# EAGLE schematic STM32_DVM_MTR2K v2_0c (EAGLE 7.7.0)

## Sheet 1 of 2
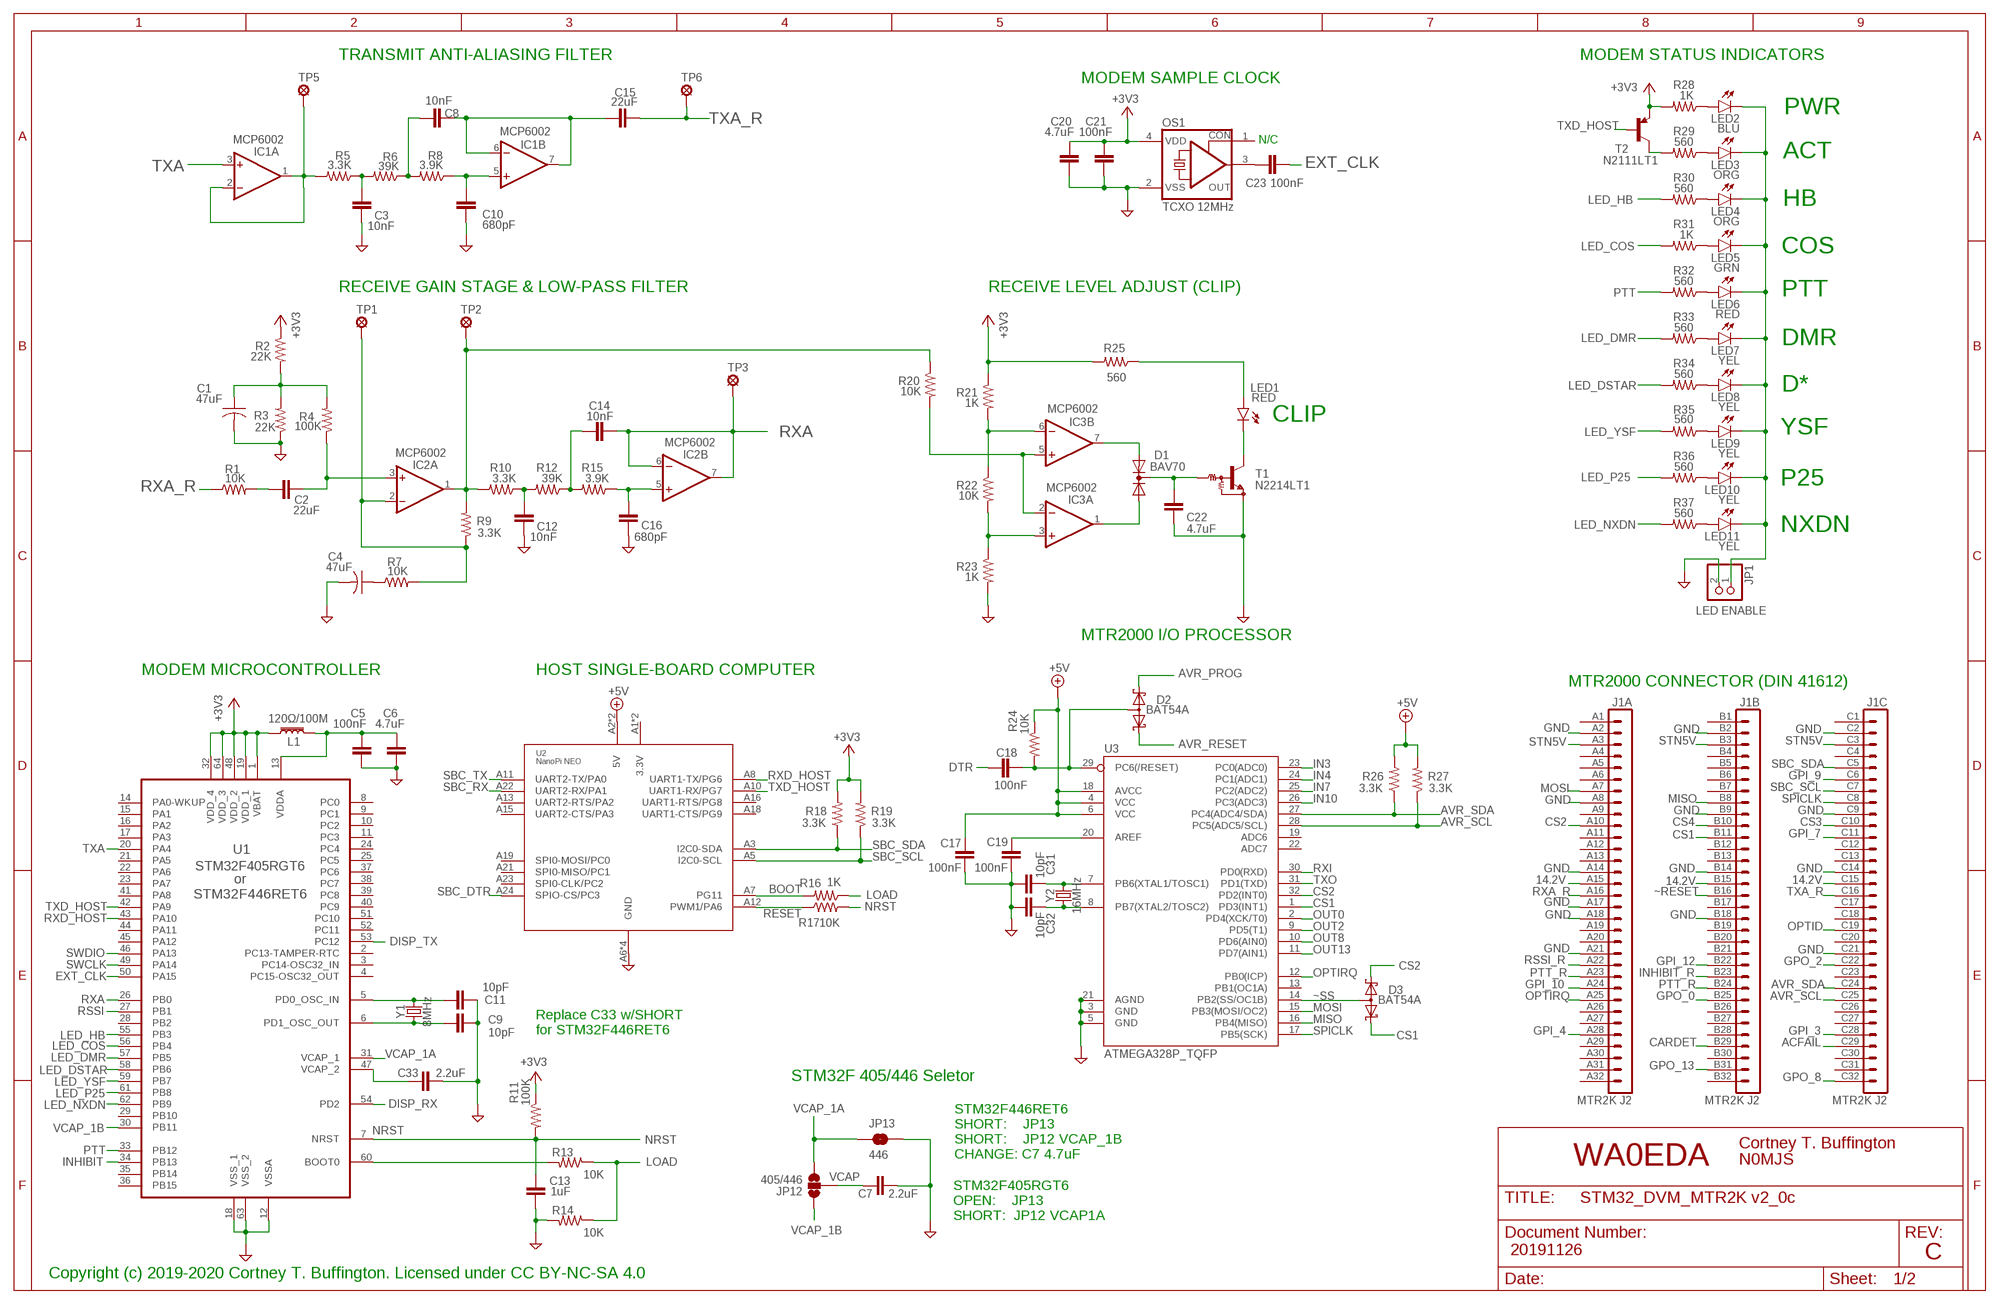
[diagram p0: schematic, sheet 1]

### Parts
C1  47uF  C-USC1210  [C1210]
C2  22uF  C-EUC1210  [C1210]
C3  10nF  C-EUC0805  [C0805]
C4  47uF  C-USC1210  [C1210]
C5  100nF  C-EUC0805  [C0805]
C6  4.7uF  C-EUC0805  [C0805]
C7  2.2uF  C-EUC0805  [C0805]
C8  10nF  C-EUC0805  [C0805]
C9  10pF  C-EUC0805  [C0805]
C10  680pF  C-EUC0805  [C0805]
C11  10pF  C-EUC0805  [C0805]
C12  10nF  C-EUC0805  [C0805]
C13  1uF  C-EUC0805  [C0805]
C14  10nF  C-EUC0805  [C0805]
C15  22uF  C-EUC1210  [C1210]
C16  680pF  C-EUC0805  [C0805]
C17  100nF  C-EUC0805  [C0805]
C18  100nF  C-EUC0805  [C0805]
C19  100nF  C-EUC0805  [C0805]
C20  4.7uF  C-EUC0805  [C0805]
C21  100nF  C-EUC0805  [C0805]
C22  4.7uF  C-EUC0805  [C0805]
C23  100nF  C-EUC0805  [C0805]
C31  10pF  C-EUC0805  [C0805]
C32  10pF  C-EUC0805  [C0805]
C33  2.2uF  C-EUC0805  [C0805]
D1  BAV70  DIODE_AC-CA_  [SOT23C]
D2  BAT54A  [SOT23]
D3  BAT54A  [SOT23]
IC1  MCP6002  TL082D  [SO08]
IC2  MCP6002  TL082D  [SO08]
IC3  MCP6002  TL082D  [SO08]
J1  MTR2K J2  VG96-3  [VG96]
JP1  LED ENABLE  PINHD-1X2  [1X02]
JP12  405/446  JUMPER-SMT_3_NO_NO-SILK  [SMT-JUMPER_3_NO_NO-SILK]
JP13  446  JUMPER-SMT_2_NO_NO-SILK  [SMT-JUMPER_2_NO_NO-SILK]
L1  120Ω/100M  FERRITE_BEAD-0603  [0603]
LED1  RED  LED0603  [LED-0603]
LED2  BLU  LED0603  [LED-0603]
LED3  ORG  LED0603  [LED-0603]
LED4  ORG  LED0603  [LED-0603]
LED5  GRN  LED0603  [LED-0603]
LED6  RED  LED0603  [LED-0603]
LED7  YEL  LED0603  [LED-0603]
LED8  YEL  LED0603  [LED-0603]
LED9  YEL  LED0603  [LED-0603]
LED10  YEL  LED0603  [LED-0603]
LED11  YEL  LED0603  [LED-0603]
OS1  TCXO 12MHz  OSC-OE-CFPS-9  [5.2X3.4-4-PAD]
R1  10K  R-US_R0805  [R0805]
R2  22K  R-US_R0805  [R0805]
R3  22K  R-US_R0805  [R0805]
R4  100K  R-US_R0805  [R0805]
R5  3.3K  R-US_R0805  [R0805]
R6  39K  R-US_R0805  [R0805]
R7  10K  R-US_R0805  [R0805]
R8  3.9K  R-US_R0805  [R0805]
R9  3.3K  R-US_R0805  [R0805]
R10  3.3K  R-US_R0805  [R0805]
R11  100K  R-US_R0805  [R0805]
R12  39K  R-US_R0805  [R0805]
R13  10K  R-US_R0805  [R0805]
R14  10K  R-US_R0805  [R0805]
R15  3.9K  R-US_R0805  [R0805]
R16  1K  R-US_R0805  [R0805]
R17  10K  R-US_R0805  [R0805]
R18  3.3K  R-US_R0805  [R0805]
R19  3.3K  R-US_R0805  [R0805]
R20  10K  R-US_R0805  [R0805]
R21  1K  R-US_R0805  [R0805]
R22  10K  R-US_R0805  [R0805]
R23  1K  R-US_R0805  [R0805]
R24  10K  R-US_R0805  [R0805]
R25  560  R-US_R0805  [R0805]
R26  3.3K  R-US_R0805  [R0805]
R27  3.3K  R-US_R0805  [R0805]
R28  1K  R-US_R0805  [R0805]
R29  560  R-US_R0805  [R0805]
R30  560  R-US_R0805  [R0805]
R31  1K  R-US_R0805  [R0805]
R32  560  R-US_R0805  [R0805]
R33  560  R-US_R0805  [R0805]
R34  560  R-US_R0805  [R0805]
R35  560  R-US_R0805  [R0805]
R36  560  R-US_R0805  [R0805]
R37  560  R-US_R0805  [R0805]
T1  N2214LT1  MUN2211T1-NPN_DRIVER-SC59-BEC  [SC59-BEC]
T2  N2111LT1  MMUN2111LT1-PNP-SC59-BEC  [SC59-BEC]
TP1  MCS10B  [MCS10B]
TP2  MCS10B  [MCS10B]
TP3  MCS10B  [MCS10B]
TP5  MCS10B  [MCS10B]
TP6  MCS10B  [MCS10B]
U1  STM32F405RGT6  [QFP50P1200X1200X160-64N]
U2  NanoPi NEO  NANOPI-NEO_MINIMALMINIMAL  [NANOPI-NEO]
U3  ATMEGA328P_TQFP  [TQFP32-08]
Y1  8MHz  CRYSTALSMD-3.2X2.5  [CRYSTAL-SMD-3.2X2.5MM]
Y2  16MHz  CRYSTALSMD-3.2X2.5  [CRYSTAL-SMD-3.2X2.5MM]

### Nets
14.2V: J1.A15 J1.B15 J1.C15 ; also sheet 2
+3V3: C20.2 C21.2 L1.1 OS1.4(VDD) R2.1 R11.1 R18.2 R19.2 R21.1 R25.2 R28.2 T2.E U1.1(VBAT) U1.19(VDD_1) U1.32(VDD_4) U1.48(VDD_2) U1.64(VDD_3) ; also sheet 2
+5V: C17.2 R24.1 R26.2 R27.2 U2.A2(5V) U2.A4(5V) U3.4(VCC) U3.6(VCC) U3.18(AVCC) ; also sheet 2
ACFAIL: J1.C29
AREF: C19.2 U3.20(AREF)
AVR_PROG: D2.1(K1) ; also sheet 2
AVR_RESET: D2.2(K2) ; also sheet 2
AVR_SCL: J1.C25 R27.1 U3.28(PC5(ADC5/SCL))
AVR_SDA: J1.C24 R26.1 U3.27(PC4(ADC4/SDA))
BOOT: R16.2 U2.A7(PG11) ; also sheet 2
BOOT0: R13.2 U1.60(BOOT0)
CARDET: J1.B29
CS1: D3.2(K2) J1.B11 U3.1(PD3(INT1))
CS2: D3.1(K1) J1.A10 U3.32(PD2(INT0))
CS3: J1.C10
CS4: J1.B10
DISP_RX: U1.54(PD2) ; also sheet 2
DISP_TX: U1.53(PC12) ; also sheet 2
DTR: C18.2 ; also sheet 2
EXT_CLK: C23.2 U1.50(PA15)
GND: C1.2 C3.2 C4.2 C5.1 C6.1 C7.1 C9.2 C10.2 C11.2 C12.2 C13.2 C16.2 C17.1 C19.1 C20.1 C21.1 C22.2 C31.2 C32.2 C33.1 J1.A2 J1.A8 J1.A14 J1.A17 J1.A18 J1.A21 J1.B2 J1.B9 J1.B14 J1.B18 J1.C2 J1.C9 J1.C14 J1.C21 JP1.2 JP13.2 OS1.2(VSS) R3.1 R14.2 R23.2 T1.E U1.12(VSSA) U1.18(VSS_1) U1.63(VSS_2) U2.A6(GND) U2.A9(GND) U2.A14(GND) U2.A20(GND) U3.3(GND) U3.5(GND) U3.21(AGND) ; also sheet 2
GPI_3: J1.C28 ; also sheet 2
GPI_4: J1.A28 ; also sheet 2
GPI_7: J1.C11 ; also sheet 2
GPI_9: J1.C6
GPI_10: J1.A24 ; also sheet 2
GPI_12: J1.B22
GPO_0: J1.B25 ; also sheet 2
GPO_2: J1.C22 ; also sheet 2
GPO_8: J1.C32 ; also sheet 2
GPO_13: J1.B31 ; also sheet 2
IN3: U3.23(PC0(ADC0)) ; also sheet 2
IN4: U3.24(PC1(ADC1)) ; also sheet 2
IN7: U3.25(PC2(ADC2)) ; also sheet 2
IN10: U3.26(PC3(ADC3)) ; also sheet 2
INHIBIT: U1.34(PB13) ; also sheet 2
INHIBIT_R: J1.B23 ; also sheet 2
LED_COS: R31.2 U1.56(PB4)
LED_DMR: R33.2 U1.57(PB5)
LED_DSTAR: R34.2 U1.58(PB6)
LED_HB: R30.2 U1.55(PB3)
LED_NXDN: R37.2 U1.62(PB9)
LED_P25: R36.2 U1.61(PB8)
LED_YSF: R35.2 U1.59(PB7)
LOAD: R13.1 R14.1 R16.1 ; also sheet 2
MISO: J1.B8 U3.16(PB4(MISO)) ; also sheet 2
MOSI: J1.A7 U3.15(PB3(MOSI/OC2)) ; also sheet 2
N$1: C23.1 OS1.3(OUT)
N$2: C2.2 R1.2
N$5: C4.1 R7.1
N$10: C8.2 C15.2 IC1.6(B:-IN) IC1.7(B:OUT)
N$11: C11.1 U1.5(PD0_OSC_IN) Y1.3
N$12: C9.1 U1.6(PD1_OSC_OUT) Y1.1
N$17: IC1.1(A:OUT) IC1.2(A:-IN) R5.2 TP5.MP
N$19: IC2.1(A:OUT) R9.2 R10.2 R20.1 TP2.MP
N$21: IC2.2(A:-IN) R7.2 R9.1 TP1.MP
N$24: C8.1 R6.1 R8.2
N$25: C10.1 IC1.5(B:+IN) R8.1
N$26: C3.1 R5.1 R6.2
N$28: C2.1 IC2.3(A:+IN) R4.1
N$29: C1.1 R2.2 R3.2 R4.2
N$30: LED2.A R28.1
N$33: LED3.A R29.1
N$34: LED4.A R30.1
N$38: R29.2 T2.C
N$40: LED7.A R33.1
N$41: C14.1 R12.1 R15.2
N$42: C16.1 IC2.5(B:+IN) R15.1
N$43: C12.1 R10.1 R12.2
N$44: LED8.A R34.1
N$45: LED9.A R35.1
N$46: LED10.A R36.1
N$51: LED5.A R31.1
N$52: LED6.A R32.1
N$54: IC3.6(B:-IN) R21.2 R22.1
N$55: IC3.3(A:+IN) R22.2 R23.1
N$56: JP1.1 LED2.C LED3.C LED4.C LED5.C LED6.C LED7.C LED8.C LED9.C LED10.C LED11.C
N$57: LED1.A R25.1
N$58: LED1.C T1.C
N$59: IC3.2(A:-IN) IC3.5(B:+IN) R20.2
N$60: D1.2(A2) IC3.7(B:OUT)
N$61: D1.1(A1) IC3.1(A:OUT)
N$63: C22.1 D1.3(K) T1.B
N$65: LED11.A R37.1
NRST: C13.1 R11.2 R17.2 U1.7(NRST) ; also sheet 2
OPTID: J1.C19 ; also sheet 2
OPTIRQ: J1.A25 U3.12(PB0(ICP))
OUT0: U3.2(PD4(XCK/T0)) ; also sheet 2
OUT2: U3.9(PD5(T1)) ; also sheet 2
OUT8: U3.10(PD6(AIN0)) ; also sheet 2
OUT13: U3.11(PD7(AIN1)) ; also sheet 2
PTT: R32.2 U1.33(PB12) ; also sheet 2
PTT_R: J1.A23 J1.B24 ; also sheet 2
RESET: R17.1 U2.A12(PWM1/PA6) ; also sheet 2
RSSI: U1.27(PB1) ; also sheet 2
RSSI_R: J1.A22 ; also sheet 2
RST: C18.1 D2.3(AA) R24.2 U3.29(PC6(/RESET)) ; also sheet 2
RXA: C14.2 IC2.6(B:-IN) IC2.7(B:OUT) TP3.MP U1.26(PB0)
RXA_R: J1.A16 R1.1
RXD_HOST: U1.43(PA10) U2.A8(UART1-TX/PG6) ; also sheet 2
RXI: U3.30(PD0(RXD)) ; also sheet 2
SBC_DTR: U2.A24(SPIO-CS/PC3) ; also sheet 2
SBC_RX: U2.A22(UART2-RX/PA1) ; also sheet 2
SBC_SCL: J1.C7 R19.1 U2.A5(I2C0-SCL)
SBC_SDA: J1.C5 R18.1 U2.A3(I2C0-SDA)
SBC_TX: U2.A11(UART2-TX/PA0) ; also sheet 2
SPICLK: J1.C8 U3.17(PB5(SCK)) ; also sheet 2
STN5V: J1.A3 J1.B3 J1.C3 ; also sheet 2
SWCLK: U1.49(PA14) ; also sheet 2
SWDIO: U1.46(PA13) ; also sheet 2
TXA: IC1.3(A:+IN) U1.20(PA4)
TXA_R: C15.1 J1.C16 TP6.MP
TXD_HOST: T2.B U1.42(PA9) U2.A10(UART1-RX/PG7) ; also sheet 2
TXO: U3.31(PD1(TXD)) ; also sheet 2
VCAP: C7.2 JP12.2
VCAP_1A: JP12.3 JP13.1 U1.31(VCAP_1)
VCAP_1B: JP12.1 U1.30(PB11)
VCAP_2: C33.2 U1.47(VCAP_2)
VDDA: C5.2 C6.2 L1.2 U1.13(VDDA)
XTAL1: C31.1 U3.7(PB6(XTAL1/TOSC1)) Y2.3
XTAL2: C32.1 U3.8(PB7(XTAL2/TOSC2)) Y2.1
~RESET: J1.B16 ; also sheet 2
~SS: D3.3(AA) U3.14(PB2(SS/OC1B))
Unconnected: J1.A1 J1.A4 J1.A5 J1.A6 J1.A9 J1.A11 J1.A12 J1.A13 J1.A19 J1.A20 J1.A26 J1.A27 J1.A29 J1.A30 J1.A31 J1.A32 J1.B1 J1.B4 J1.B5 J1.B6 J1.B7 J1.B12 J1.B13 J1.B17 J1.B19 J1.B20 J1.B21 J1.B26 J1.B27 J1.B28 J1.B30 J1.B32 J1.C1 J1.C4 J1.C12 J1.C13 J1.C17 J1.C18 J1.C20 J1.C23 J1.C26 J1.C27 J1.C30 J1.C31 OS1.1(CON) U1.2(PC13-TAMPER-RTC) U1.3(PC14-OSC32_IN) U1.4(PC15-OSC32_OUT) U1.8(PC0) U1.9(PC1) U1.10(PC2) U1.11(PC3) U1.14(PA0-WKUP) U1.15(PA1) U1.16(PA2) U1.17(PA3) U1.21(PA5) U1.22(PA6) U1.23(PA7) U1.24(PC4) U1.25(PC5) U1.28(PB2) U1.29(PB10) U1.35(PB14) U1.36(PB15) U1.37(PC6) U1.38(PC7) U1.39(PC8) U1.40(PC9) U1.41(PA8) U1.44(PA11) U1.45(PA12) U1.51(PC10) U1.52(PC11) U2.A1(3.3V) U2.A13(UART2-RTS/PA2) U2.A15(UART2-CTS/PA3) U2.A16(UART1-RTS/PG8) U2.A17(3.3V) U2.A18(UART1-CTS/PG9) U2.A19(SPI0-MOSI/PC0) U2.A21(SPI0-MISO/PC1) U2.A23(SPI0-CLK/PC2) U3.13(PB1(OC1A)) U3.19(ADC6) U3.22(ADC7)

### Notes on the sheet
- TRANSMIT ANTI-ALIASING FILTER | MODEM STATUS INDICATORS
- MODEM SAMPLE CLOCK
- PWR
- N/C
- ACT
- HB
- COS
- RECEIVE GAIN STAGE & LOW-PASS FILTER | RECEIVE LEVEL ADJUST (CLIP) | PTT
- DMR
- D*
- CLIP
- YSF
- P25
- NXDN
- MTR2000 I/O PROCESSOR
- MODEM MICROCONTROLLER | HOST SINGLE-BOARD COMPUTER
- MTR2000 CONNECTOR (DIN 41612)
- or
- STM32F446RET6
- Replace C33 w/SHORT
  for STM32F446RET6
- STM32F 405/446 Seletor
- Cortney T. Buffington
- STM32F446RET6
  SHORT:    JP13
  SHORT:    JP12 VCAP_1B
  CHANGE: C7 4.7uF
- WA0EDA | N0MJS
- STM32F405RGT6
  OPEN:    JP13
  SHORT:  JP12 VCAP1A
- 20191126
- C
- Copyright (c) 2019-2020 Cortney T. Buffington. Licensed under CC BY-NC-SA 4.0

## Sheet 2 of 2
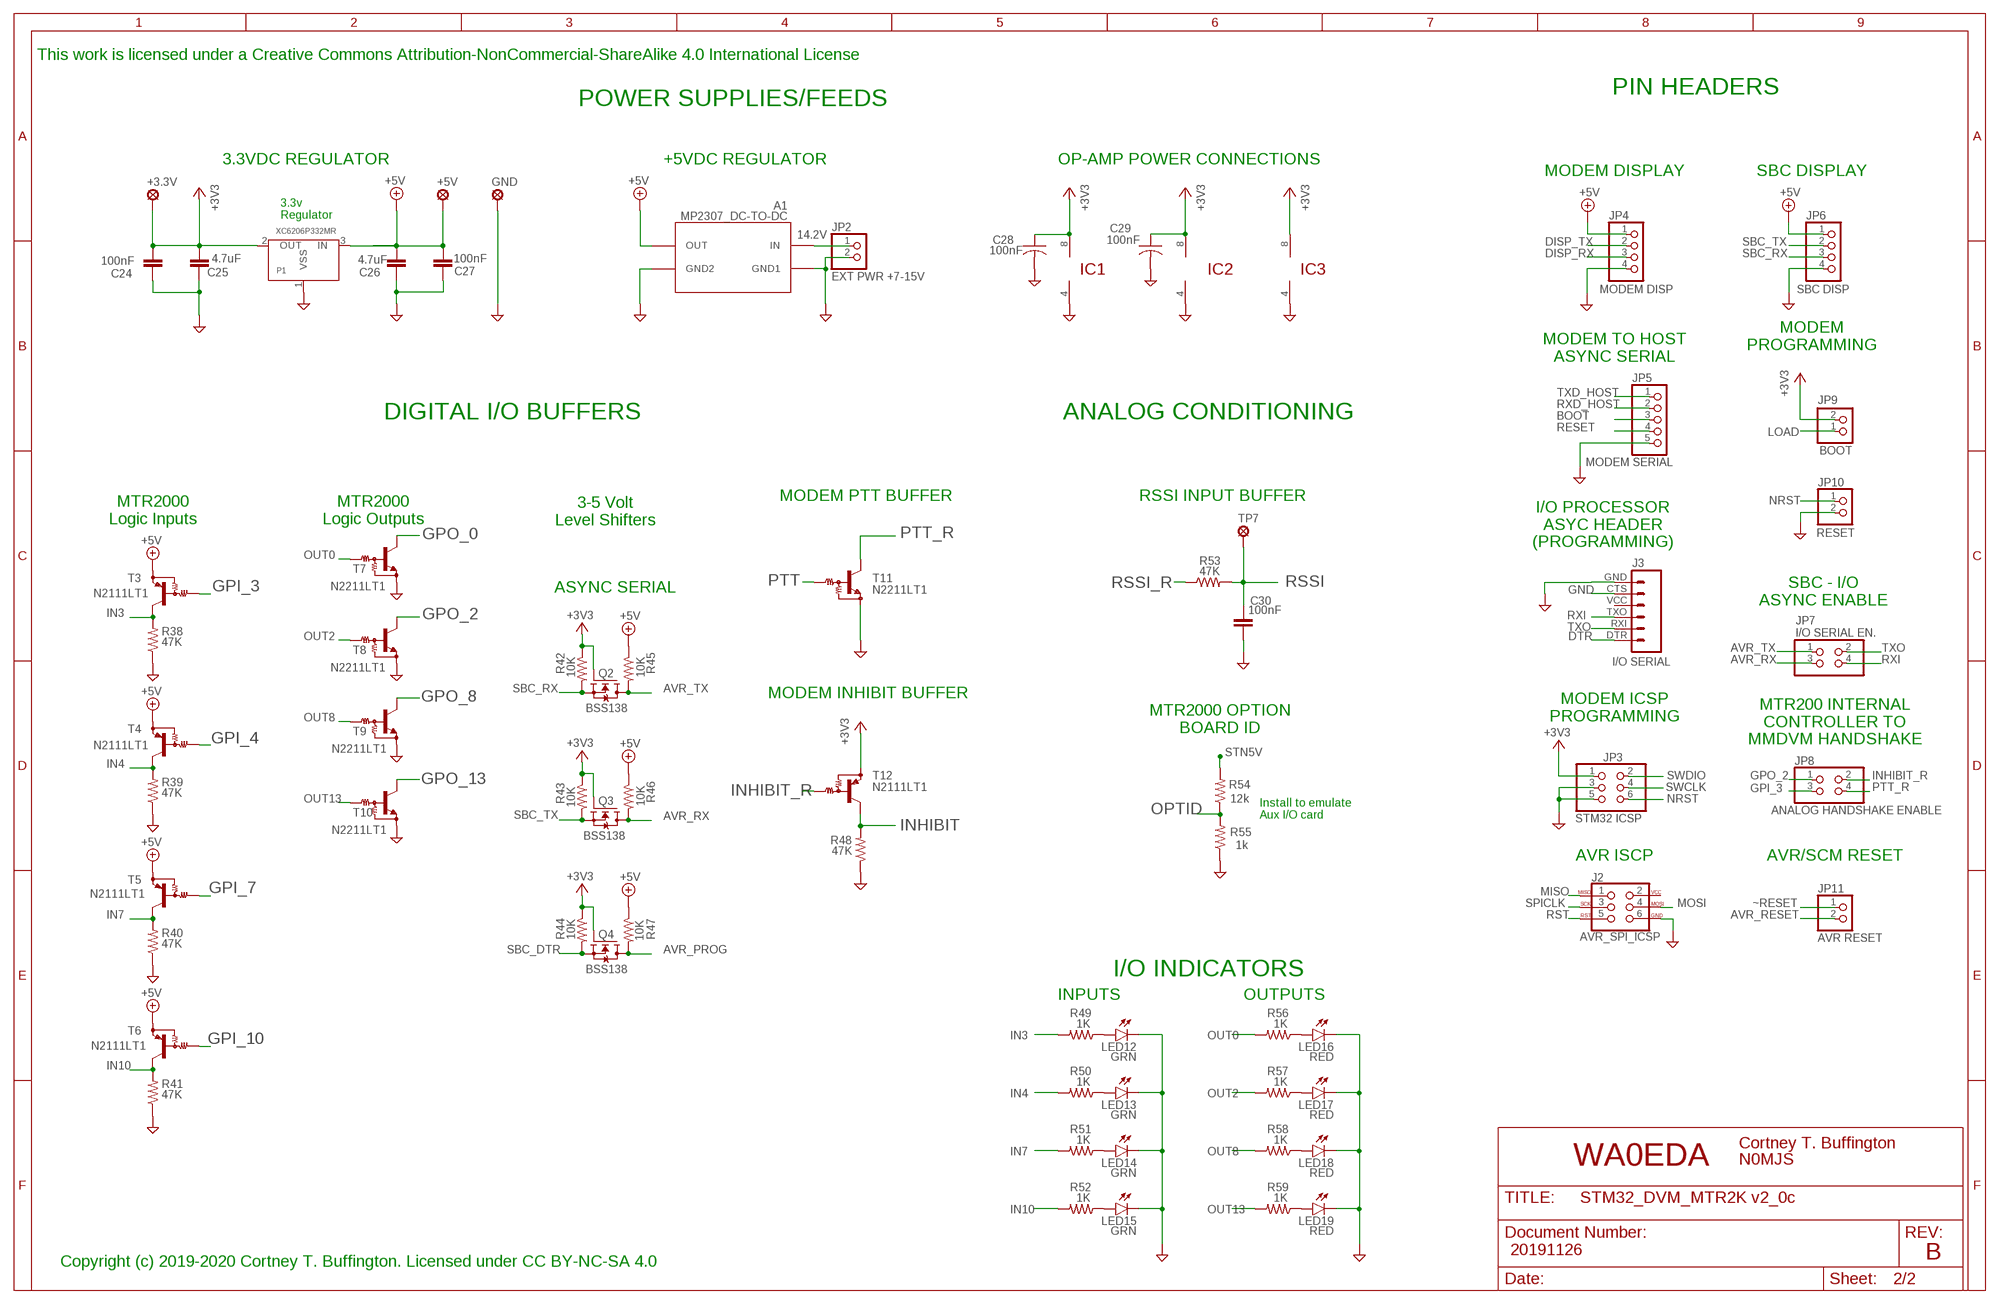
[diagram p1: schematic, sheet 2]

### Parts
+3.3V  MCS10B  [MCS10B]
+5V  MCS10B  [MCS10B]
A1  MP2307_DC-TO-DC  MPS2307_DC-TO-DC  [MPS2307_DC-TO-DC]
C24  100nF  C-EUC0805  [C0805]
C25  4.7uF  C-EUC0805  [C0805]
C26  4.7uF  C-EUC0805  [C0805]
C27  100nF  C-EUC0805  [C0805]
C28  100nF  C-USC0805  [C0805]
C29  100nF  C-USC0805  [C0805]
C30  100nF  C-EUC0805  [C0805]
GND  MCS10B  [MCS10B]
J2  AVR_SPI_ICSP  AVR_SPI_PROG_3X2PTH  [2X3]
J3  I/O SERIAL  6_PIN_SERIAL_CABLEPTH  [FTDI_BASIC]
JP2  EXT PWR +7-15V  PINHD-1X2  [1X02]
JP3  STM32 ICSP  PINHD-2X3  [2X03]
JP4  MODEM DISP  PINHD-1X4  [1X04]
JP5  MODEM SERIAL  PINHD-1X5  [1X05]
JP6  SBC DISP  PINHD-1X4  [1X04]
JP7  I/O SERIAL EN.  PINHD-2X2  [2X02]
JP8  ANALOG HANDSHAKE ENABLE  PINHD-2X2  [2X02]
JP9  BOOT  PINHD-1X2/90  [1X02/90]
JP10  RESET  PINHD-1X2/90  [1X02/90]
JP11  AVR RESET  PINHD-1X2  [1X02]
LED12  GRN  LED0603  [LED-0603]
LED13  GRN  LED0603  [LED-0603]
LED14  GRN  LED0603  [LED-0603]
LED15  GRN  LED0603  [LED-0603]
LED16  RED  LED0603  [LED-0603]
LED17  RED  LED0603  [LED-0603]
LED18  RED  LED0603  [LED-0603]
LED19  RED  LED0603  [LED-0603]
P1  XC6206P332MR  XC6206SOT-23  [XC6206_SOT-23]
Q2  BSS138  [SOT23]
Q3  BSS138  [SOT23]
Q4  BSS138  [SOT23]
R38  47K  R-US_R0805  [R0805]
R39  47K  R-US_R0805  [R0805]
R40  47K  R-US_R0805  [R0805]
R41  47K  R-US_R0805  [R0805]
R42  10K  R-US_R0805  [R0805]
R43  10K  R-US_R0805  [R0805]
R44  10K  R-US_R0805  [R0805]
R45  10K  R-US_R0805  [R0805]
R46  10K  R-US_R0805  [R0805]
R47  10K  R-US_R0805  [R0805]
R48  47K  R-US_R0805  [R0805]
R49  1K  R-US_R0805  [R0805]
R50  1K  R-US_R0805  [R0805]
R51  1K  R-US_R0805  [R0805]
R52  1K  R-US_R0805  [R0805]
R53  47K  R-US_R0805  [R0805]
R54  12k  R-US_R0805  [R0805]
R55  1k  R-US_R0805  [R0805]
R56  1K  R-US_R0805  [R0805]
R57  1K  R-US_R0805  [R0805]
R58  1K  R-US_R0805  [R0805]
R59  1K  R-US_R0805  [R0805]
T3  N2111LT1  MUN2111LT1-PNP_DRIVER-  [SOT23-BEC]
T4  N2111LT1  MUN2111LT1-PNP_DRIVER-  [SOT23-BEC]
T5  N2111LT1  MUN2111LT1-PNP_DRIVER-  [SOT23-BEC]
T6  N2111LT1  MUN2111LT1-PNP_DRIVER-  [SOT23-BEC]
T7  N2211LT1  MUN2211T1-NPN_DRIVER-SC59-BEC  [SC59-BEC]
T8  N2211LT1  MUN2211T1-NPN_DRIVER-SC59-BEC  [SC59-BEC]
T9  N2211LT1  MUN2211T1-NPN_DRIVER-SC59-BEC  [SC59-BEC]
T10  N2211LT1  MUN2211T1-NPN_DRIVER-SC59-BEC  [SC59-BEC]
T11  N2211LT1  MUN2211T1-NPN_DRIVER-SC59-BEC  [SC59-BEC]
T12  N2111LT1  MUN2111LT1-PNP_DRIVER-  [SOT23-BEC]
TP7  MCS10B  [MCS10B]

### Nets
14.2V: A1.IN JP2.1 ; also sheet 1
+3V3: +3.3V.MP C24.2 C25.2 C28.1 C29.1 IC1.8(P:V+) IC2.8(P:V+) IC3.8(P:V+) JP3.1 JP9.2 P1.2(OUT) Q2.1(G) Q3.1(G) Q4.1(G) R42.1 R43.1 R44.1 T12.E ; also sheet 1
+5V: +5V.MP A1.OUT C26.2 C27.2 JP4.1 JP6.1 P1.3(IN) R45.1 R46.1 R47.1 T3.E T4.E T5.E T6.E ; also sheet 1
AVR_PROG: Q4.3(D) R47.2 ; also sheet 1
AVR_RESET: JP11.2 ; also sheet 1
AVR_RX: JP7.3 Q3.3(D) R46.2
AVR_TX: JP7.1 Q2.3(D) R45.2
BOOT: JP5.3 ; also sheet 1
DISP_RX: JP4.3 ; also sheet 1
DISP_TX: JP4.2 ; also sheet 1
DTR: J3.DTR ; also sheet 1
GND: A1.GND1 A1.GND2 C24.1 C25.1 C26.1 C27.1 C28.2 C29.2 C30.1 GND.MP IC1.4(P:V-) IC2.4(P:V-) IC3.4(P:V-) J2.6 J3.CTS J3.GND JP2.2 JP3.3 JP3.5 JP4.4 JP5.5 JP6.4 JP10.2 LED12.C LED13.C LED14.C LED15.C LED16.C LED17.C LED18.C LED19.C P1.1(VSS) R38.1 R39.1 R40.1 R41.1 R48.1 R55.1 T7.E T8.E T9.E T10.E T11.E ; also sheet 1
GPI_3: JP8.3 T3.B ; also sheet 1
GPI_4: T4.B ; also sheet 1
GPI_7: T5.B ; also sheet 1
GPI_10: T6.B ; also sheet 1
GPO_0: T7.C ; also sheet 1
GPO_2: JP8.1 T8.C ; also sheet 1
GPO_8: T9.C ; also sheet 1
GPO_13: T10.C ; also sheet 1
IN3: R38.2 R49.2 T3.C ; also sheet 1
IN4: R39.2 R50.2 T4.C ; also sheet 1
IN7: R40.2 R51.2 T5.C ; also sheet 1
IN10: R41.2 R52.2 T6.C ; also sheet 1
INHIBIT: R48.2 T12.C ; also sheet 1
INHIBIT_R: JP8.2 T12.B ; also sheet 1
LOAD: JP9.1 ; also sheet 1
MISO: J2.1 ; also sheet 1
MOSI: J2.4 ; also sheet 1
N$4: LED16.A R56.1
N$8: LED12.A R49.1
N$13: LED17.A R57.1
N$14: LED13.A R50.1
N$15: LED18.A R58.1
N$16: LED14.A R51.1
N$18: LED19.A R59.1
N$20: LED15.A R52.1
NRST: JP3.6 JP10.1 ; also sheet 1
OPTID: R54.1 R55.2 ; also sheet 1
OUT0: R56.2 T7.B ; also sheet 1
OUT2: R57.2 T8.B ; also sheet 1
OUT8: R58.2 T9.B ; also sheet 1
OUT13: R59.2 T10.B ; also sheet 1
PTT: T11.B ; also sheet 1
PTT_R: JP8.4 T11.C ; also sheet 1
RESET: JP5.4 ; also sheet 1
RSSI: C30.2 R53.2 TP7.MP ; also sheet 1
RSSI_R: R53.1 ; also sheet 1
RST: J2.5 ; also sheet 1
RXD_HOST: JP5.2 ; also sheet 1
RXI: J3.TXO JP7.4 ; also sheet 1
SBC_DTR: Q4.2(S) R44.2 ; also sheet 1
SBC_RX: JP6.3 Q2.2(S) R42.2 ; also sheet 1
SBC_TX: JP6.2 Q3.2(S) R43.2 ; also sheet 1
SPICLK: J2.3 ; also sheet 1
STN5V: R54.2 ; also sheet 1
SWCLK: JP3.4 ; also sheet 1
SWDIO: JP3.2 ; also sheet 1
TXD_HOST: JP5.1 ; also sheet 1
TXO: J3.RXI JP7.2 ; also sheet 1
~RESET: JP11.1 ; also sheet 1
Unconnected: J2.2 J3.VCC

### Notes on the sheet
- This work is licensed under a Creative Commons Attribution-NonCommercial-ShareAlike 4.0 International License
- PIN HEADERS
- POWER SUPPLIES/FEEDS
- 3.3VDC REGULATOR | +5VDC REGULATOR | OP-AMP POWER CONNECTIONS
- MODEM DISPLAY | SBC DISPLAY
- 3.3v
  Regulator
- IC1 | IC2 | IC3
- MODEM
  PROGRAMMING
- MODEM TO HOST
  ASYNC SERIAL
- DIGITAL I/O BUFFERS | ANALOG CONDITIONING
- MODEM PTT BUFFER | RSSI INPUT BUFFER
- MTR2000
  Logic Inputs
- MTR2000
  Logic Outputs
- 3-5 Volt
  Level Shifters
- I/O PROCESSOR
  ASYC HEADER
  (PROGRAMMING)
- ASYNC SERIAL
- SBC - I/O
  ASYNC ENABLE
- MODEM INHIBIT BUFFER
- MODEM ICSP
  PROGRAMMING
- MTR2000 OPTION
  BOARD ID
- MTR200 INTERNAL
  CONTROLLER TO
  MMDVM HANDSHAKE
- Install to emulate
  Aux I/O card
- AVR ISCP | AVR/SCM RESET
- I/O INDICATORS
- INPUTS | OUTPUTS
- Cortney T. Buffington
- WA0EDA | N0MJS
- 20191126
- B
- Copyright (c) 2019-2020 Cortney T. Buffington. Licensed under CC BY-NC-SA 4.0

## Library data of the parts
+3.3V +5V GND TP1-TP3 TP5-TP7 = solpad:MCS10B: SOLDER PAD
A1 = Custom:MPS2307_DC-TO-DC: MP2307 DC-to-DC Buck Regulator
C1 C4 C28 C29 = rcl:C-US: CAPACITOR, American symbol
C2 C3 C5-C27 C30-C33 = rcl:C-EU: CAPACITOR, European symbol
D1 = semicon-smd-ipc:DIODE_AC-CA_: DUAL DIODE
D2 D3 = diode:BAT54A: Schottky Diodes Source: Fairchild .. BAT54.pdf
IC1-IC3 = linear:TL082: OP AMP Data sheet; DATA_SHEET: <a href="http://www.ti.com/lit/ds/symlink/tl084a.pdf"> Data sheet </a>
J1 = 19inch:VG96-3: PCB EUROCARD, 96-pin type C/ABC, 2.54 mm
J2 = SparkFun-Connectors:AVR_SPI_PROG_3X2: AVR ISP 6 Pin This is the reduced ISP connector for AVR programming. Common on Arduino. This footprint will take up less PCB space and can be used with a 10-pin to 6-pin adapter such as SKU: BOB-08508 **Special note about "TEST_POINT" package. The stop mask is on the top side, so if you want your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
J3 = SparkFun-Connectors:6_PIN_SERIAL_CABLE: 6-pin header connection for use with the "FTDI BASIC" pinout - CABLE SIDE. Also known as "Arduino Serial Program Header". This is used on a design to provide a 6-pin connection point for serial communication usually from a USB cable (D+/D-) to these headers (RX/TX). It also has the remaining pins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
JP1 JP2 JP9-JP11 = pinhead:PINHD-1X2: PIN HEADER
JP3 = pinhead:PINHD-2X3: PIN HEADER
JP4 JP6 = pinhead:PINHD-1X4: PIN HEADER
JP5 = pinhead:PINHD-1X5: PIN HEADER
JP7 JP8 = pinhead:PINHD-2X2: PIN HEADER
JP12 = SparkFun-Jumpers:JUMPER-SMT_3_NO: Normally open jumper This jumper has three pads in close proximity to each other. Apply solder to close the connection(s).
JP13 = SparkFun-Jumpers:JUMPER-SMT_2_NO: Normally open jumper
L1 = SparkFun-Coils:FERRITE_BEAD: Ferrite Bead (blocks, cores, rings, chokes, etc.); PROD_ID: NDUC-13805; VALUE: 30Ω/1.8A
LED1-LED19 = SparkFun-LED:LED: LED (Generic)
OS1 = Custom:OSC-OE: OSCILLATOR WITH OE
P1 = Voltage Regulator:XC6206: XC6206P , linear regulator. Producted by TOREX.Co Store Information: EXCEL device corporation http://www.excel-d.com/access/index.html
Q2-Q4 = bss138_10:BSS138: BSS138 N-Channel Logic Level Enhancement Mode Field Effect Transistor Source: http://www.fairchildsemi.com/datasheets/BS/BSS138.pdf; MF: Fairchild; MPN: BSS138; OC_FARNELL: 9845330; OC_NEWARK: 67R2009
R1-R59 = rcl:R-US_: RESISTOR, American symbol
T1 T7-T11 = transistor:*-NPN_DRIVER-: NPN Bias Resistor Transistor
T2 = transistor:*-PNP-: PNP Transistror
T3-T6 T12 = transistor:*-PNP_DRIVER-: PNP Bias Resistor Transistor
U1 = STM32F4xx-CTB:STM32F405RGT6
U2 = NanoPi:NANOPI-NEO_MINIMAL
U3 = SparkFun-IC-Microcontroller:ATMEGA328P_TQFP: Popular 328P in QFP Storefront component: ATmega328 - TQFP (COM-13448) Datasheet SparkFun Products SparkFun RedBoard - Programmed with Arduino (DEV-12757) Arduino Pro Mini 328 - 5V/16MHz (DEV-11113) Arduino Pro Mini 328 - 3.3V/8MHz (DEV-11114) SparkFun OpenLog (DEV-13712) SparkFun MicroView - OLED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; PROD_ID: IC-09069
Y1 Y2 = SparkFun-Clocks:CRYSTAL: Crystals (Generic)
